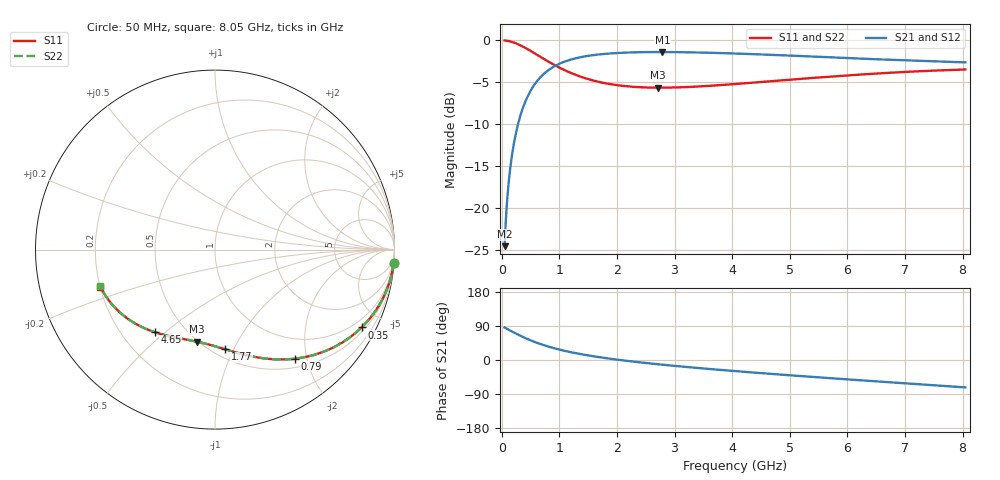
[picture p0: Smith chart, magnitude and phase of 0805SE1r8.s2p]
! AVX Thin Film Operation		Date: August 2001
! Description: Accu-P® Series, Thin Film, SMD, RF Capacitor
! Part Number: 08051J1R8ABT
! 50 MHz  -  8.05 GHz
! Serial Measurements
# mhz S db R 50
!	S11		S21		S12		S22
!	dB	Phase	dB	Phase	dB	Phase	dB	Phase
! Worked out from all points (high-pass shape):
!   401 points, 50 MHz to 8.05 GHz, reference 50 ohm
!   highest |S21| = -1.39 dB at 2.79 GHz (marker M1); lowest = -24.5 dB at 50 MHz (marker M2)
!   |S21| within 3 dB of the highest: 671.3 MHz to end of sweep
!   lowest |S11| = -5.6 dB at 2.71 GHz (marker M3), VSWR 3.19, Z = 24.6 - j34.8 ohm
!   |S11| at or under -10 dB: nowhere
!   |S22| runs from -5.6 to 0.0 dB; largest |S21 - S12| = 0
!   S11 on the Smith chart (normalised r, x): 50 MHz: 1, -27; 350 MHz: 0.65, -3.91; 790 MHz: 0.64, -1.80; 1.77 GHz: 0.57, -0.93; 4.65 GHz: 0.34, -0.46; 8.05 GHz: 0.20, -0.15
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50  -0.02 -4.2  -24.49 85.8  -24.49 85.8  -0.02 -4.2
70  -0.03 -5.9  -21.59 84.1  -21.59 84.1  -0.03 -5.9
130  -0.10 -10.9  -16.30 79.1  -16.30 79.1  -0.10 -10.9
170  -0.17 -14.2  -14.05 75.8  -14.05 75.8  -0.17 -14.2
250  -0.37 -20.5  -10.93 69.5  -10.93 69.5  -0.37 -20.5
350  -0.68 -28.0  -8.39 62.0  -8.39 62.0  -0.68 -28.0
450  -1.05 -34.8  -6.67 55.1  -6.67 55.1  -1.05 -34.9
550  -1.46 -41.1  -5.45 48.9  -5.45 48.9  -1.46 -41.1
790  -2.45 -53.7  -3.65 36.3  -3.65 36.3  -2.45 -53.7
1070  -3.48 -65.0  -2.59 25.0  -2.59 25.0  -3.48 -65.0
1390  -4.37 -74.9  -1.98 15.0  -1.98 15.0  -4.37 -75.0
1770  -5.07 -84.2  -1.62 5.7  -1.62 5.7  -5.07 -84.3
2190  -5.48 -92.5  -1.45 -2.6  -1.45 -2.6  -5.48 -92.6
2710  -5.63 -101.1  -1.39 -11.2  -1.39 -11.2  -5.63 -101.2
2730  -5.63 -101.4  -1.39 -11.5  -1.39 -11.5  -5.63 -101.5
2790  -5.63 -102.3  -1.39 -12.4  -1.39 -12.4  -5.63 -102.4
3390  -5.50 -110.8  -1.44 -20.9  -1.44 -20.9  -5.50 -110.9
4050  -5.20 -119.2  -1.57 -29.3  -1.57 -29.3  -5.20 -119.2
4650  -4.88 -126.2  -1.72 -36.4  -1.72 -36.4  -4.88 -126.3
5390  -4.48 -134.5  -1.93 -44.6  -1.93 -44.6  -4.48 -134.5
6730  -3.86 -148.6  -2.31 -58.7  -2.31 -58.7  -3.86 -148.7
8050  -3.47 -162.1  -2.62 -72.3  -2.62 -72.3  -3.47 -162.2
